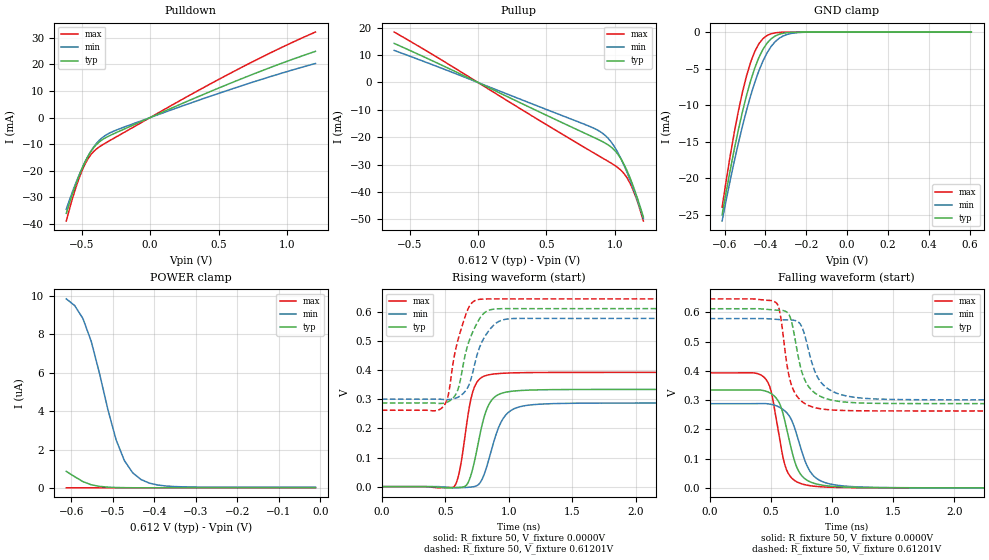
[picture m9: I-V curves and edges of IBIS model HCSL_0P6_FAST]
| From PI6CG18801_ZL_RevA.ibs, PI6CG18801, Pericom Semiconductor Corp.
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|   Model HCSL_OUT
[Model]   HCSL_0P6_FAST
Model_type Output
Vref=0.6000V
Vmeas=900mV
| variable   typ   min   max
C_comp   2.000pF   1.970pF   2.030pF
[Voltage Range]   0.61201V   0.57834V   0.64563V
[POWER Clamp Reference]   0.61201V   0.57834V   0.64563V
[GND Clamp Reference]   0.0000V   0.0000V   0.0000V
[Pullup Reference]   0.61201V   0.57834V   0.64563V
[Pulldown Reference]   0.0000V   0.0000V   0.0000V
[Temperature Range]   25   85   -40
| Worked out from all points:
|   slope of the pulldown table from 0 to 0.092 V, typ, clamps not added: 43.8 ohm
|   slope of the pullup table from 0 to 0.092 V, typ, clamps not added: 41.4 ohm
|   GND clamp passes 1 mA (typ) near -0.37 V on its own axis
|   falling waveform, R_fixture 50, V_fixture 0.0000V: 20-80 % time 126ps typ, 148ps min, 105ps max; typ from 0.334 V to 0 V
|   rising waveform, R_fixture 50, V_fixture 0.0000V: 20-80 % time 109ps typ, 132ps min, 86.1ps max; typ from 0 V to 0.334 V
|   falling waveform, R_fixture 50, V_fixture 0.61201V: 20-80 % time 118ps typ, 142ps min, 93.7ps max; typ from 0.612 V to 0.288 V
|   rising waveform, R_fixture 50, V_fixture 0.61201V: 20-80 % time 121ps typ, 129ps min, 111ps max; typ from 0.288 V to 0.612 V
[GND Clamp]
| Voltage   I(typ)   I(min)   I(max)
-612mV    -25.02mA   -25.88mA   -24mA
-572mV    -18.86mA   -20.25mA   -16.88mA
-552mV    -16mA      -17.64mA   -13.68mA
-512mV    -10.87mA   -12.84mA   -8.188mA
-492mV    -8.627mA   -10.67mA   -5.955mA
-452mV    -4.921mA   -6.891mA   -2.659mA
-432mV    -3.494mA   -5.314mA   -1.606mA
-392mV    -1.518mA   -2.854mA   -474.6uA
-372mV    -924.8uA   -1.975mA   -235.2uA
-332mV    -299.3uA   -841.7uA   -49.75uA
-252mV    -21.66uA   -107.3uA   -1.344uA
608mV     1.088nA    32.69nA    -5.916pA
[POWER Clamp]
| Voltage   I(typ)   I(min)   I(max)
-612mV    861nA      9.857uA    1.622nA
-592mV    584.2nA    9.512uA    621.3pA
-572mV    326.3nA    8.835uA    247.2pA
-552mV    161.3nA    7.648uA    107.3pA
-512mV    36.25nA    4.099uA    34.37pA
-492mV    17.5nA     2.503uA    26.17pA
-472mV    8.826nA    1.419uA    22.47pA
-452mV    4.814nA    782.1nA    20.43pA
-432mV    2.956nA    432.9nA    19.01pA
-392mV    1.685nA    147.6nA    16.72pA
-352mV    1.395nA    67.95nA    14.59pA
-12.01mV  1.099nA    32.4nA     -3.301pA
[Pulldown]
| Voltage   I(typ)   I(min)   I(max)
-612mV    -36.03mA   -34.49mA   -38.92mA
-572mV    -29.56mA   -28.64mA   -31.37mA
-532mV    -23.7mA    -23.29mA   -24.78mA
-492mV    -18.59mA   -18.51mA   -19.38mA
-472mV    -16.38mA   -16.35mA   -17.2mA
-432mV    -12.73mA   -12.62mA   -13.91mA
-392mV    -10.14mA   -9.725mA   -11.83mA
-312mV    -7.227mA   -6.264mA   -9.161mA
27.99mV   641.2uA    526.5uA    828.2uA
568mV     12.54mA    10.27mA    16.19mA
908mV     19.41mA    15.88mA    25.08mA
1.208V    24.93mA    20.36mA    32.2mA
[Pullup]
| Voltage   I(typ)   I(min)   I(max)
-612mV    14.27mA    11.7mA     18.42mA
-272mV    6.49mA     5.323mA    8.39mA
768mV     -18.25mA   -15.07mA   -23.43mA
908mV     -21.57mA   -18.47mA   -27.55mA
968mV     -23.42mA   -21.41mA   -29.33mA
1.008V    -25.33mA   -24.4mA    -30.61mA
1.048V    -28.19mA   -28.22mA   -32.24mA
1.088V    -32.14mA   -32.77mA   -34.75mA
1.108V    -34.49mA   -35.27mA   -36.51mA
1.148V    -39.84mA   -40.66mA   -41.16mA
1.168V    -42.79mA   -43.54mA   -44.01mA
1.208V    -49.14mA   -49.69mA   -50.59mA
[Falling Waveform]
R_fixture = 50
V_fixture = 0.0000V
V_fixture_min = 0.0000V
V_fixture_max = 0.0000V
|   Time   V(typ)   V(min)   V(max)
0s        334.3mV    287.6mV    392.9mV
450ps     331.4mV    287.9mV    375.6mV
500ps     322.7mV    285.5mV    333.4mV
560ps     297.1mV    277.6mV    197.8mV
630ps     200.4mV    256.7mV    60.28mV
710ps     72.56mV    184.1mV    21.11mV
800ps     25.02mV    71.84mV    8.814mV
940ps     7.927mV    18.36mV    2.873mV
1.24ns    1.17mV     2.779mV    405.1uV
5ns       17.26uV    18.47uV    16.17uV
[Rising Waveform]
R_fixture = 50
V_fixture = 0.0000V
V_fixture_min = 0.0000V
V_fixture_max = 0.0000V
|   Time   V(typ)   V(min)   V(max)
0s        8.072uV    8.706uV    8.005uV
570ps     -3.349mV   -3.912mV   -304.1uV
620ps     -2.119mV   -3.712mV   68.75mV
670ps     6.338mV    -2.654mV   217.2mV
720ps     66.71mV    -524.7uV   329.7mV
790ps     211mV      24.67mV    376.2mV
850ps     286.8mV    102.8mV    385.1mV
970ps     324mV      242.4mV    390.1mV
1.18ns    332.1mV    281.2mV    392.2mV
5ns       334.3mV    287.6mV    392.9mV
[Falling Waveform]
R_fixture = 50
V_fixture = 0.61201V
V_fixture_min = 0.57834V
V_fixture_max = 0.64563V
|   Time   V(typ)   V(min)   V(max)
0s        612mV      578.3mV    645.6mV
550ps     607.2mV    575.6mV    630mV
580ps     607mV      574.8mV    585.3mV
640ps     597mV      573.8mV    400.1mV
680ps     548.5mV    573.1mV    338.6mV
770ps     376.3mV    531.8mV    290.1mV
890ps     316mV      372.5mV    271.4mV
1.06ns    295.3mV    320.2mV    264.8mV
1.38ns    288.7mV    303.3mV    262.9mV
5ns       287.8mV    300.7mV    262.7mV
[Rising Waveform]
R_fixture = 50
V_fixture = 0.61201V
V_fixture_min = 0.57834V
V_fixture_max = 0.64563V
|   Time   V(typ)   V(min)   V(max)
0s        287.7mV    300.6mV    262.7mV
480ps     286.5mV    299.8mV    273mV
520ps     291.2mV    299.2mV    306.7mV
590ps     322.9mV    305.3mV    486mV
650ps     437.6mV    323.8mV    575.2mV
700ps     514mV      364.8mV    626.4mV
760ps     569.4mV    465.3mV    643.1mV
880ps     610.1mV    554.2mV    645.4mV
1.02ns    612mV      577.6mV    645.4mV
5ns       612mV      578.3mV    645.6mV
[Ramp]
| variable   typ   min   max
dV/dt_r   0.20057V/108.67p   0.17248V/131.80p   0.23574V/86.131p
dV/dt_f   0.19444V/117.52p   0.16672V/142.33p   0.22791V/93.840p
R_load = 50
